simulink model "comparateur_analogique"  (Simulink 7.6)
settings: Solver=ode45  StartTime=0.0  StopTime=1  RelTol=1e-3
undefined symbols (not defined in the file or in its folder): sigbuilder_block
libraries: fl_lib x12, nesl_utility x3

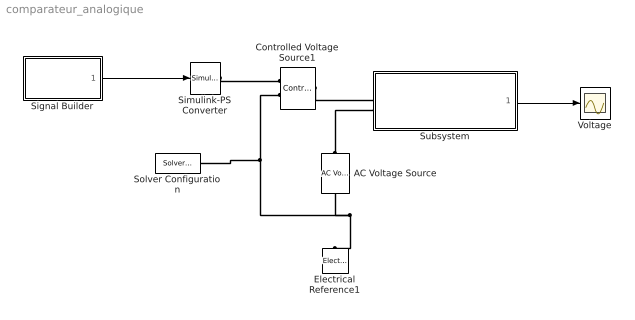
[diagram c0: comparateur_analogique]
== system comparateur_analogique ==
  AC Voltage Source : fl_lib/Electrical/Electrical Sources/AC Voltage Source  DialogController=NetworkEngine.DynNeDlgSource  SystemSampleTime=-1  amp=1 V  shift=0 rad  omega=1 Hz  i_Log=off  v_Log=off  LocalVarNames=|current|voltage|power  LocalVarDescs=|Current (A)|Voltage (V)|Power (W)  LocalVarLogging=[0 0 0]
  Controlled Voltage Source1 : fl_lib/Electrical/Electrical Sources/Controlled Voltage Source  DialogController=NetworkEngine.DynNeDlgSource  SystemSampleTime=-1  i_Log=off  v_Log=off  LocalVarNames=|current|voltage|power  LocalVarDescs=|Current (A)|Voltage (V)|Power (W)  LocalVarLogging=[0 0 0]
  Electrical Reference1 : fl_lib/Electrical/Electrical Elements/Electrical Reference  DialogController=NetworkEngine.DynNeDlgSource  SystemSampleTime=-1  i_Log=off  LocalVarNames=|i  LocalVarDescs=|i  LocalVarLogging=[]
  Signal Builder : Subsystem  Tag=STV Subsys  LoadFcn=sigbuilder_block('load');  StartFcn=sigbuilder_block('start');  StopFcn=sigbuilder_block('stop');  ClipboardFcn=sigbuilder_block('clipboard');
  Simulink-PS Converter : nesl_utility/Simulink-PS Converter  DialogController=NetworkEngine.DynNeUtilDlgSource  SystemSampleTime=-1  PhysicalDomain=network_engine_domain  LeftPortType=input  RightPortType=output  SubClassName=ps_input  Unit=1  AffineConversion=off  InputFilterTimeConstant=.001  UdotUserProvided=0
  Solver Configuration : nesl_utility/Solver Configuration  DialogController=NetworkEngine.DynNeUtilDlgSource  SystemSampleTime=-1  PhysicalDomain=network_engine_domain  LeftPortType=input  RightPortType=generic  SubClassName=solver  Accelerate=off  Profile=off  ResidualTolerance=1e-9  MaxNonlinIter=12  MaxModeIter=2  DoFixedCost=off  UseLocalSampling=off  DoDC=off  LinearAlgebra=Sparse  LocalSolverSampleTime=.001  LocalSolverChoice=NE_BACKWARD_EULER_ADVANCER  UseLocalSolver=off
  Subsystem : Subsystem
  Voltage : Scope
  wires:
  Subsystem/1(v1-v2) -> Voltage/1
  Signal Builder/1(Signal 2) -> Simulink-PS Converter/1
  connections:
  AC Voltage Source/LConn1 -- Subsystem/LConn2
  Controlled Voltage Source1/RConn2 -- AC Voltage Source/RConn1 -- Electrical Reference1/LConn1 -- Solver Configuration/RConn1
  Controlled Voltage Source1/LConn1 -- Subsystem/LConn1
  Simulink-PS Converter/RConn1 -- Controlled Voltage Source1/RConn1

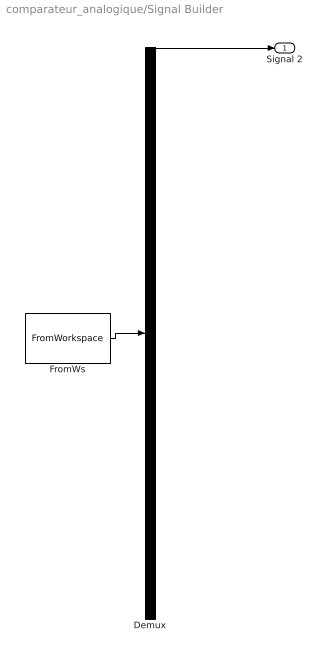
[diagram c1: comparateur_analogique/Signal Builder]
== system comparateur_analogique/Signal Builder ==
  Demux : Demux  Tag=STV Demux  Outputs=1
  FromWs : FromWorkspace  Tag=STV FromWs  VariableName=tuvar  SampleTime=0  SigBuilderData=DataTag0  VnvData=DataTag1
  Signal 2 : Outport  Tag=STV Outport
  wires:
  Demux/1 -> Signal 2/1
  FromWs/1 -> Demux/1

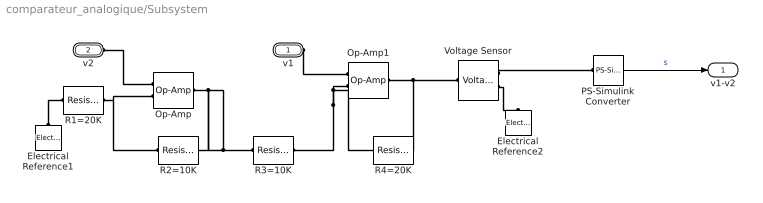
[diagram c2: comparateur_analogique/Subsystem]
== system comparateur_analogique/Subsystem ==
  Electrical Reference1 : fl_lib/Electrical/Electrical Elements/Electrical Reference  DialogController=NetworkEngine.DynNeDlgSource  SystemSampleTime=-1  i_Log=off  LocalVarNames=|i  LocalVarDescs=|i  LocalVarLogging=[]
  Electrical Reference2 : fl_lib/Electrical/Electrical Elements/Electrical Reference  DialogController=NetworkEngine.DynNeDlgSource  SystemSampleTime=-1  i_Log=off  LocalVarNames=|i  LocalVarDescs=|i  LocalVarLogging=[]
  Op-Amp : fl_lib/Electrical/Electrical Elements/Op-Amp  DialogController=NetworkEngine.DynNeDlgSource  SystemSampleTime=-1  i1_Log=off  v1_Log=off  outI_Log=off  LocalVarNames=|i1|v1|outI  LocalVarDescs=|i1|v1|outI  LocalVarLogging=[]
  Op-Amp1 : fl_lib/Electrical/Electrical Elements/Op-Amp  DialogController=NetworkEngine.DynNeDlgSource  SystemSampleTime=-1  i1_Log=off  v1_Log=off  outI_Log=off  LocalVarNames=|i1|v1|outI  LocalVarDescs=|i1|v1|outI  LocalVarLogging=[]
  PS-Simulink Converter : nesl_utility/PS-Simulink Converter  DialogController=NetworkEngine.DynNeUtilDlgSource  SystemSampleTime=-1  PhysicalDomain=network_engine_domain  LeftPortType=input  RightPortType=output  SubClassName=ps_output  Unit=1  AffineConversion=off
  R1=20K : fl_lib/Electrical/Electrical Elements/Resistor  DialogController=NetworkEngine.DynNeDlgSource  SystemSampleTime=-1  R=20e3 Ohm  i_Log=off  v_Log=off  LocalVarNames=|current|voltage|power  LocalVarDescs=|Resistor current (A)|Voltage across resistor (V)|Power (W)  LocalVarLogging=[0 0 0]
  R2=10K : fl_lib/Electrical/Electrical Elements/Resistor  DialogController=NetworkEngine.DynNeDlgSource  SystemSampleTime=-1  R=10e3 Ohm  i_Log=off  v_Log=off  LocalVarNames=|current|voltage|power  LocalVarDescs=|Resistor current (A)|Voltage across resistor (V)|Power (W)  LocalVarLogging=[0 0 0]
  R3=10K : fl_lib/Electrical/Electrical Elements/Resistor  DialogController=NetworkEngine.DynNeDlgSource  SystemSampleTime=-1  R=10e3 Ohm  i_Log=off  v_Log=off  LocalVarNames=|current|voltage|power  LocalVarDescs=|Resistor current (A)|Voltage across resistor (V)|Power (W)  LocalVarLogging=[0 0 0]
  R4=20K : fl_lib/Electrical/Electrical Elements/Resistor  DialogController=NetworkEngine.DynNeDlgSource  SystemSampleTime=-1  R=20e3 Ohm  i_Log=off  v_Log=off  LocalVarNames=|current|voltage|power  LocalVarDescs=|Resistor current (A)|Voltage across resistor (V)|Power (W)  LocalVarLogging=[0 0 0]
  Voltage Sensor : fl_lib/Electrical/Electrical Sensors/Voltage Sensor  DialogController=NetworkEngine.DynNeDlgSource  SystemSampleTime=-1  i1_Log=off  v1_Log=off  LocalVarNames=|i1|v1  LocalVarDescs=|i1|v1  LocalVarLogging=[]
  v1 : PMIOPort  Port=1  Side=Left
  v2 : PMIOPort  Port=2  Side=Left
  v1-v2 : Outport
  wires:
  PS-Simulink Converter/1 -> v1-v2/1  "s"
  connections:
  Electrical Reference1/LConn1 -- R1=20K/LConn1
  Voltage Sensor/RConn2 -- Electrical Reference2/LConn1
  R1=20K/RConn1 -- R2=10K/LConn1 -- Op-Amp/LConn2
  Op-Amp/RConn1 -- R2=10K/RConn1 -- R3=10K/LConn1
  Op-Amp1/LConn2 -- R4=20K/LConn1 -- R3=10K/RConn1
  Op-Amp1/RConn1 -- Voltage Sensor/LConn1 -- R4=20K/RConn1
  Voltage Sensor/RConn1 -- PS-Simulink Converter/LConn1
  v1/RConn1 -- Op-Amp1/LConn1
  v2/RConn1 -- Op-Amp/LConn1
